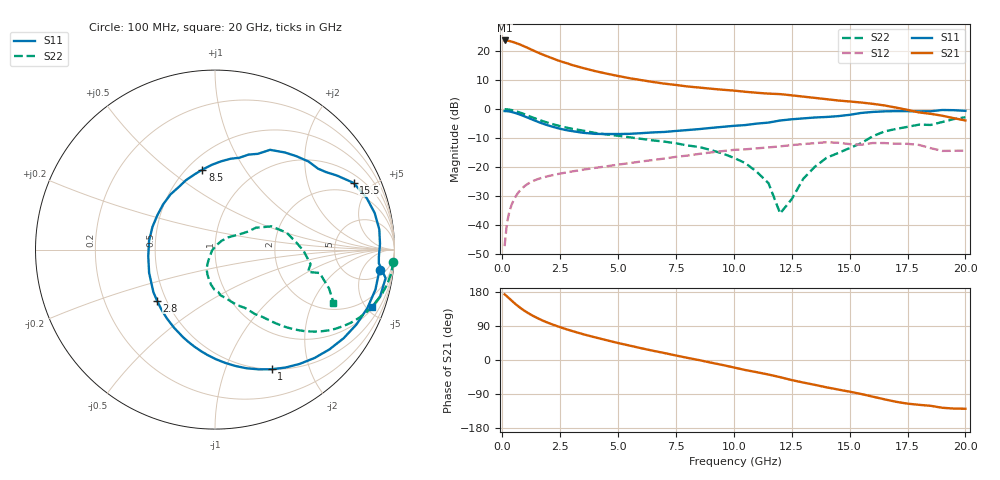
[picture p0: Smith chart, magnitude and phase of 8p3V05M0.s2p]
! Infineon Technologies  Discrete & RF Semiconductors
! BFP640
! VCE =  3.0 V,  IC =  5.0 mA
! Common Emitter S-Parameters:  Sep 2002
# GHz  S  MA  R  50
!  f  S11  S21  S12  S22
! GHz  MAG  ANG  MAG  ANG  MAG  ANG  MAG  ANG
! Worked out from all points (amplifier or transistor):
!   59 points, 100 MHz to 20 GHz, reference 50 ohm
!   highest |S21| = 23.7 dB at 100 MHz (marker M1)
!   |S21| within 3 dB of that: start of sweep to 1.213 GHz
!   unconditionally stable (mu >= 1): 4.724 GHz to 11.06 GHz
!   at 1 GHz: K = 0.29, MSG = 23.9 dB, |S12| = -26.4 dB
!   at 5.5 GHz: K = 1.05, MAG = 13.3 dB, |S12| = -18.7 dB
!   at 20 GHz: K = 0.99, MSG = 5.2 dB, |S12| = -14.3 dB
!   lowest NFmin = 0.36 dB at 900 MHz
!   S11 on the Smith chart (normalised r, x): 100 MHz: 8, -12; 1 GHz: 0.50, -1.46; 2.8 GHz: 0.45, -0.31; 8.5 GHz: 0.59, +0.66; 15.5 GHz: 1.40, +3.91; 20 GHz: 1.13, -5.47
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0.1  0.9237 -6.9  15.29 173.2  0.0043 80.5  0.9961 -3.9
0.2  0.9212 -14.0  15.22 168.0  0.0107 83.0  0.9904 -7.8
0.3  0.9094 -21.0  14.97 162.5  0.0166 80.2  0.9779 -11.6
0.5  0.8702 -34.6  14.21 151.4  0.0273 73.0  0.9388 -18.9
0.6  0.846 -41.1  13.77 146.2  0.0321 69.5  0.9143 -22.3
0.8  0.7929 -53.4  12.82 136.6  0.0407 63.1  0.8598 -28.3
1  0.7375 -64.7  11.84 128.3  0.048 57.5  0.8022 -33.4
1.4  0.634 -84.8  10.01 114.2  0.0589 48.8  0.6948 -41.0
1.8  0.5521 -102.1  8.565 102.6  0.0666 42.8  0.6103 -46.1
2.2  0.4917 -117.6  7.42 93.0  0.0727 38.6  0.5462 -49.7
2.8  0.4301 -138.7  6.168 80.6  0.0809 34.0  0.476 -53.7
3.5  0.3891 -160.7  5.096 67.9  0.0901 30.0  0.4238 -58.1
5  0.3708 160.0  3.722 44.8  0.1098 22.4  0.3467 -65.8
7  0.4029 120.1  2.748 18.4  0.1399 12.0  0.2742 -78.1
8.5  0.451 99.0  2.352 -0.3  0.1683 2.3  0.2219 -91.1
10.5  0.5297 75.1  1.987 -26.5  0.202 -15.6  0.1165 -113.8
11.5  0.5845 65.9  1.848 -38.4  0.2179 -23.4  0.0523 -126.3
12  0.6349 61.1  1.811 -45.3  0.2272 -26.5  0.0158 -168.4
13.5  0.7156 43.3  1.559 -65.6  0.2577 -42.0  0.101 42.7
15.5  0.8569 25.7  1.297 -89.7  0.242 -62.3  0.2581 28.2
17  0.9222 7.0  1.062 -110.2  0.2526 -79.7  0.4537 5.2
20  0.932 -19.9  0.636 -128.7  0.1917 -99.9  0.7231 -24.1
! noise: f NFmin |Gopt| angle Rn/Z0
0.9  0.36  0.37  21  0.14
1.8  0.65  0.15  30  0.11
2.4  0.72  0.18  59  0.12
3  0.83  0.14  115  0.11
4  0.93  0.08  -161  0.1
5  1.07  0.17  -86  0.15
6  1.26  0.25  -114  0.13
